PROGRAM MAIN
VAR
	//输入
	start AT%I* : BOOL;                     //启动按钮
	limit_switch_up  AT%I*:BOOL;               //上限位
	limit_switch_down AT%I*:BOOL;             //下限位
	//输出
	solenoid_valve_up AT%Q*:BOOL;             //上行电磁阀
	solenoid_valve_down AT%Q*:BOOL;           //下行电磁阀
	//延时
	delayed_time: TON;                        //下限位延时功能块
END_VAR

IF start THEN  
   solenoid_valve_down:=TRUE;                 //控制下行电磁阀吸合，气缸下行 
   solenoid_valve_up:=FALSE;                                                                                 
END_IF
IF limit_switch_down THEN                //触发下限位，下行电磁阀松开
   solenoid_valve_down:=FALSE;
END_IF
delayed_time(IN:= limit_switch_down  , PT:=T#3S , Q=> , ET=> );

IF delayed_time.Q  THEN 
   solenoid_valve_up:=TRUE;                   //控制上行电磁阀吸合，气缸上行  
   solenoid_valve_down:=FALSE;                                                                                        
END_IF
IF limit_switch_UP THEN                //触发下限位，下行电磁阀松开
   solenoid_valve_UP:=FALSE;  
END_IF


































































(*CASE state OF
	0://初始位
	  move_distance:=0;      //HMI气缸在初始位
	  work_state_light:=FALSE;//工作灯熄灭
	  limit_switch_up:=TRUE;//气缸处于上限位
	  state:=1;
	1://气缸下行
	  IF start OR solenoid_valve_down AND NOT pause THEN
	  work_state_light:=TRUE;
	  solenoid_valve_down:=TRUE;//下行电磁阀吸合，气缸下行	
	  solenoid_valve_up:=FALSE;
	  move_distance:=move_distance+0.5;
	  END_IF
	  IF move_distance>=250 THEN
		 move_distance:=250;
		 limit_switch_down:=TRUE;
		 solenoid_valve_down:=FALSE;
		 state:=2;
	   END_IF
	   
	2://下限位延时
      delayed_time(IN:=NOT delayed_time.Q  , PT:=T#3S , Q=> , ET=> );//下限位触发延时
      IF  delayed_time.Q THEN
		  limit_switch_down:=FALSE;
		  state:=3; 
	  END_IF
		 
	3://气缸上行
	IF NOT pause THEN
	  solenoid_valve_up:=TRUE;  //上行电磁阀吸合，气缸上行
	  move_distance:=move_distance-0.5;//HMI气缸上行
	END_IF
	IF move_distance<=0 THEN
		 //move_distance:=0;
		// limit_switch_up:=TRUE;//气缸到达上限位
		 //work_state_light:=FALSE;//工作状态指示灯熄灭
		 state:=0;
    END_IF
END_CASE
// 确保气缸在上下限位之间时不会限位信号不会被触发
IF move_distance>10 AND move_distance <240  THEN	
   limit_switch_up:=FALSE;
   limit_switch_down:=FALSE;
END_IF *)

END_PROGRAM
